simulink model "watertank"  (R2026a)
settings: Solver=ode3  StopTime=1200  FixedStep=parSys.Ta  MaxStep=parSys.Ta  EnableMultiTasking=on
undefined symbols (not defined in the file or in its folder): parSys, sigbuilder_block
libraries: simulink x3

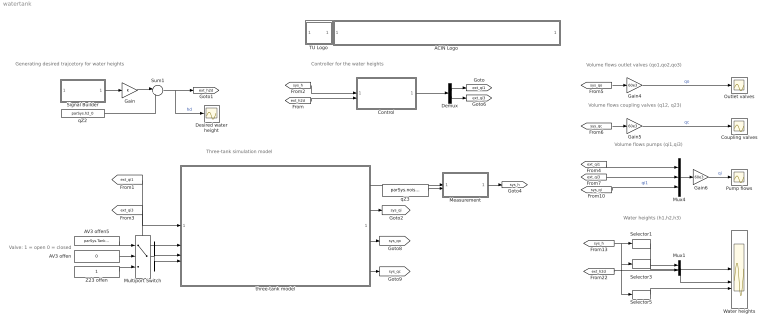
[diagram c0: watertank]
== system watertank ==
  note: Generating desired trajcetory for water heights
  note: Valve: 1 = open 0 = closed
  note: Volume flows outlet valves (qo1,qo2,qo3)
  note: Water heights (h1,h2,h3)
  note: Volume flows coupling valves (q12, q23)
  note: Volume flows pumps (qi1,qi3)
  note: Controller for the water heights
  note: Three-tank simulation model
  ACIN Logo : Subsystem
      mask init:
      | s = get_param(gcb,'UserData');
  AV3 offen : Constant  Value=0
  AV3 offen5 : Constant  Value=parSys.Tank3_on
  Control : Subsystem
  Coupling valves : Scope
  Demux : Demux  Outputs=2
  Desired water height : Scope
  Gain : Gain
  Gain4 : Gain  Gain=60e3
  Gain5 : Gain  Gain=60e3
  Gain6 : Gain  Gain=60e3
  Measurement : Subsystem
  Multiport Switch : MultiPortSwitch  DataPortOrder=Zero-based contiguous  Inputs=2  zeroidx=on
  Mux1 : Mux  Inputs=2
  Mux4 : Mux  Inputs=3
  Outlet valves : Scope
  Pump flows : Scope
  Selector1 : Selector  InputPortWidth=3  IndexOptions=Index vector (dialog)  Indices=1  OutputSizes=1
  Selector3 : Selector  InputPortWidth=3  IndexOptions=Index vector (dialog)  Indices=2  OutputSizes=1
  Selector5 : Selector  InputPortWidth=3  IndexOptions=Index vector (dialog)  Indices=3  OutputSizes=1
  Signal Builder : Subsystem  Tag=STV Subsys  LoadFcn=sigbuilder_block('load');  StartFcn=sigbuilder_block('start');  StopFcn=sigbuilder_block('stop');  ClipboardFcn=sigbuilder_block('clipboard');  mask(Sigbuilder block){tuvar=[0:10]}
      mask help: Simulink:masks:SigbuilderBlock_MD
      mask init:
      | if ~strcmp(get_param(bdroot(gcbh),'SimulationStatus'),'stopped') tuvar = sigbuilder_block('maskInit'); end
  Sum1 : Sum  Inputs=|++
  TU Logo : Subsystem
      mask init:
      | s = get_param(gcb,'UserData');
  Water heights : Scope  NumInputPorts=3
  Z23 offen : Constant
  qZ2 : Constant  Value=parSys.h2_0
  qZ3 : Constant  Value=parSys.noise_on
  three-tank model : Subsystem
      mask init:
      | S = get_param(gcb,'UserData');
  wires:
  Sum1/1 -> Desired water height/1, [ext_h2d]  "hd"
  qZ2/1 -> Sum1/2
  Demux/1 -> [ext_qi1]
  Demux/2 -> [ext_qi3]
  three-tank model/4("[q12 q23]") -> [sys_qc]
  three-tank model/3("[qo1 qo2 qo3]") -> [sys_qo]
  Z23 offen/1 -> Multiport Switch/3
  three-tank model/2("[qi1 qi3]") -> [sys_qi]
  AV3 offen5/1 -> Multiport Switch/1
  Measurement/1(hmess) -> [sys_h]
  [ext_qi1] -> three-tank model/1(qi1)
  Multiport Switch/1 -> three-tank model/3(o3), three-tank model/4(23)
  qZ3/1 -> Measurement/2(noise_on)
  AV3 offen/1 -> Multiport Switch/2
  [ext_qi3] -> three-tank model/2(qi3)
  Selector5/1 -> Water heights/3
  Mux4/1 -> Gain6/1
  Mux1/1 -> Water heights/2
  Selector1/1 -> Water heights/1
  Gain5/1 -> Coupling valves/1  "qc"
  Gain6/1 -> Pump flows/1  "qi"
  Selector3/1 -> Mux1/1
  [ext_h2d] -> Mux1/2
  [sys_qc] -> Gain5/1
  [sys_h] -> Selector5/1, Selector3/1, Selector1/1
  [sys_qo] -> Gain4/1
  Gain4/1 -> Outlet valves/1  "qo"
  [sys_qi] -> Mux4/3  "qi1"
  [ext_qi3] -> Mux4/2
  [ext_qi1] -> Mux4/1
  Gain/1 -> Sum1/1
  Signal Builder/1(Signal 2) -> Gain/1
  [sys_h] -> Control/1(x)
  [ext_h2d] -> Control/2(yref)
  Control/1(u) -> Demux/1
  three-tank model/1("[h1 h2 h3]") -> Measurement/1(h)

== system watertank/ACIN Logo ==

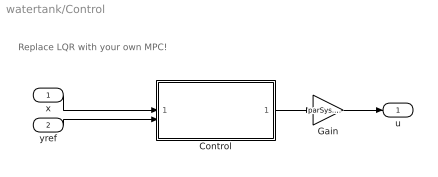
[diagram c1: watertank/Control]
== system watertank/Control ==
  note: Replace LQR with your own MPC!
  x : Inport
  yref : Inport  Port=2
  Control : MATLAB Function  TreatAsAtomicUnit=on
  Gain : Gain  Gain=parSys.qimax
  u : Outport
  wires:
  yref/1 -> Control/2(yref)
  x/1 -> Control/1(x)
  Control/1(u) -> Gain/1
  Gain/1 -> u/1

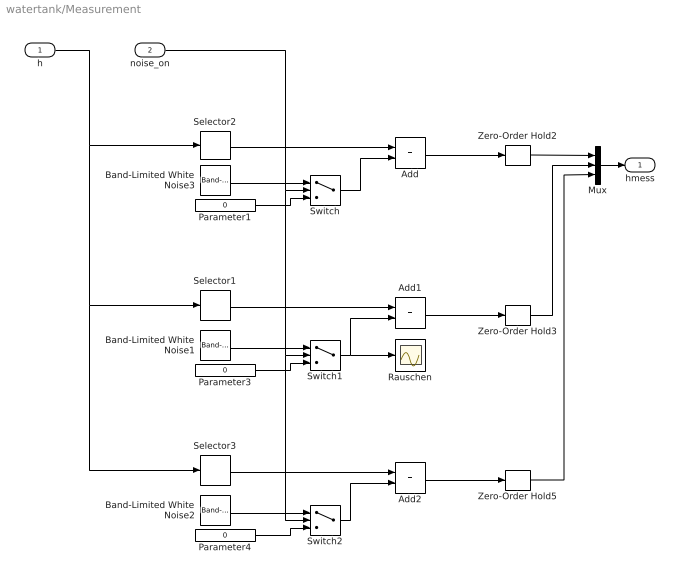
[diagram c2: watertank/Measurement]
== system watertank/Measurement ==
  h : Inport
  noise_on : Inport  Port=2
  Add : Sum
  Add1 : Sum
  Add2 : Sum
  Band-Limited White Noise1 : simulink/Sources/Band-Limited White Noise  Cov=parInit.meas.noisepow  Ts=parSys.Ts  seed=[981353]
  Band-Limited White Noise2 : simulink/Sources/Band-Limited White Noise  Cov=parInit.meas.noisepow  Ts=parSys.Ts  seed=[23343]
  Band-Limited White Noise3 : simulink/Sources/Band-Limited White Noise  Cov=parInit.meas.noisepow  Ts=parSys.Ts  seed=[23263]
  Mux : Mux  Inputs=3
  Parameter1 : Constant  Value=0  VectorParams1D=off
  Parameter3 : Constant  Value=0  VectorParams1D=off
  Parameter4 : Constant  Value=0  VectorParams1D=off
  Rauschen : Scope
  Selector1 : Selector  InputPortWidth=3  IndexOptions=Index vector (dialog)  Indices=[2]  OutputSizes=1
  Selector2 : Selector  InputPortWidth=3  IndexOptions=Index vector (dialog)  Indices=[1]  OutputSizes=1
  Selector3 : Selector  InputPortWidth=3  IndexOptions=Index vector (dialog)  Indices=[3]  OutputSizes=1
  Switch : Switch  Threshold=0.5
  Switch1 : Switch  Threshold=0.5
  Switch2 : Switch  Threshold=0.5
  Zero-Order Hold2 : ZeroOrderHold  SampleTime=parSys.Ts
  Zero-Order Hold3 : ZeroOrderHold  SampleTime=parSys.Ts
  Zero-Order Hold5 : ZeroOrderHold  SampleTime=parSys.Ts
  hmess : Outport  VectorParamsAs1DForOutWhenUnconnected=off
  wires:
  Band-Limited White Noise3/1 -> Switch/1
  Switch/1 -> Add/2
  noise_on/1 -> Switch/2, Switch1/2, Switch2/2
  Selector2/1 -> Add/1
  Parameter1/1 -> Switch/3
  Band-Limited White Noise1/1 -> Switch1/1
  Switch1/1 -> Rauschen/1, Add1/2
  Selector1/1 -> Add1/1
  Parameter3/1 -> Switch1/3
  Band-Limited White Noise2/1 -> Switch2/1
  Switch2/1 -> Add2/2
  Parameter4/1 -> Switch2/3
  Add/1 -> Zero-Order Hold2/1
  Add1/1 -> Zero-Order Hold3/1
  Add2/1 -> Zero-Order Hold5/1
  Selector3/1 -> Add2/1
  h/1 -> Selector1/1, Selector3/1, Selector2/1
  Mux/1 -> hmess/1
  Zero-Order Hold2/1 -> Mux/1
  Zero-Order Hold3/1 -> Mux/2
  Zero-Order Hold5/1 -> Mux/3

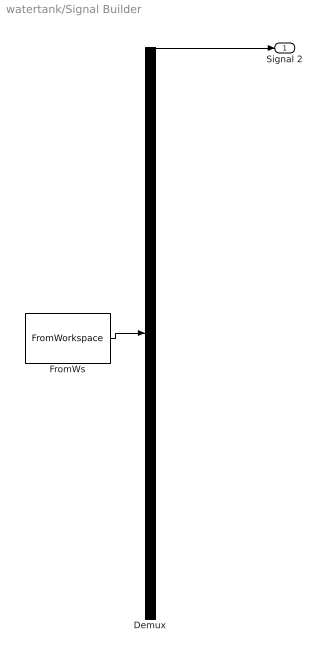
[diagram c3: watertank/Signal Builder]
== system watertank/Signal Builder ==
  Demux : Demux  Tag=STV Demux  Outputs=1
  FromWs : FromWorkspace  Tag=STV FromWs  VariableName=tuvar
  Signal 2 : Outport  Tag=STV Outport  VectorParamsAs1DForOutWhenUnconnected=off
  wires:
  FromWs/1 -> Demux/1
  Demux/1 -> Signal 2/1

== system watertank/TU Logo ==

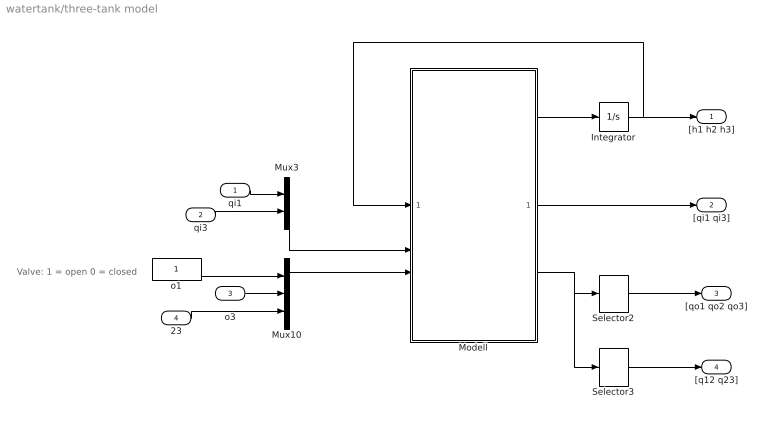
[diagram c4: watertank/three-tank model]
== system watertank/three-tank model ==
  note: Valve: 1 = open 0 = closed
  qi1 : Inport
  qi3 : Inport  Port=2
  o3 : Inport  Port=3
  23 : Inport  Port=4
  Integrator : Integrator  InitialCondition=[parSys.h1_0; parSys.h2_0; parSys.h3_0]
  Modell : MATLAB Function  TreatAsAtomicUnit=on
  Mux10 : Mux  Inputs=3
  Mux3 : Mux  Inputs=2
  Selector2 : Selector  InputPortWidth=5  IndexOptions=Index vector (dialog)  Indices=[1 2 3]  OutputSizes=1
  Selector3 : Selector  InputPortWidth=5  IndexOptions=Index vector (dialog)  Indices=[4 5]  OutputSizes=1
  o1 : Constant
  "[h1 h2 h3]" : Outport  VectorParamsAs1DForOutWhenUnconnected=off
  "[qi1 qi3]" : Outport  Port=2  VectorParamsAs1DForOutWhenUnconnected=off
  "[qo1 qo2 qo3]" : Outport  Port=3  VectorParamsAs1DForOutWhenUnconnected=off
  "[q12 q23]" : Outport  Port=4  VectorParamsAs1DForOutWhenUnconnected=off
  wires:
  o1/1 -> Mux10/1
  qi1/1 -> Mux3/1
  qi3/1 -> Mux3/2
  Selector2/1 -> "[qo1 qo2 qo3]"/1
  Selector3/1 -> "[q12 q23]"/1
  23/1 -> Mux10/3
  o3/1 -> Mux10/2
  Mux10/1 -> Modell/3(is_open)
  Modell/1(dx) -> Integrator/1
  Integrator/1 -> Modell/1(x), "[h1 h2 h3]"/1
  Mux3/1 -> Modell/2(qi)
  Modell/3(q_valve) -> Selector3/1, Selector2/1
  Modell/2(q_pump) -> "[qi1 qi3]"/1

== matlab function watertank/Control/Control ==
function u    = fcn(x, yref, parSys)
% LQR based on the linearized discrete-time dynamics

% Calculate total control input
u = parSys.uR + parSys.K * (x - parSys.xR) + parSys.G * (yref - parSys.yR);

end

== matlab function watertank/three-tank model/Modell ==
function [dx, q_pump, q_valve] = fcn(x, qi, is_open, parSys)
%#codegen

[dx, q_pump, q_valve] = watertank_mfun(x, qi, is_open, parSys);

% Function end
end
